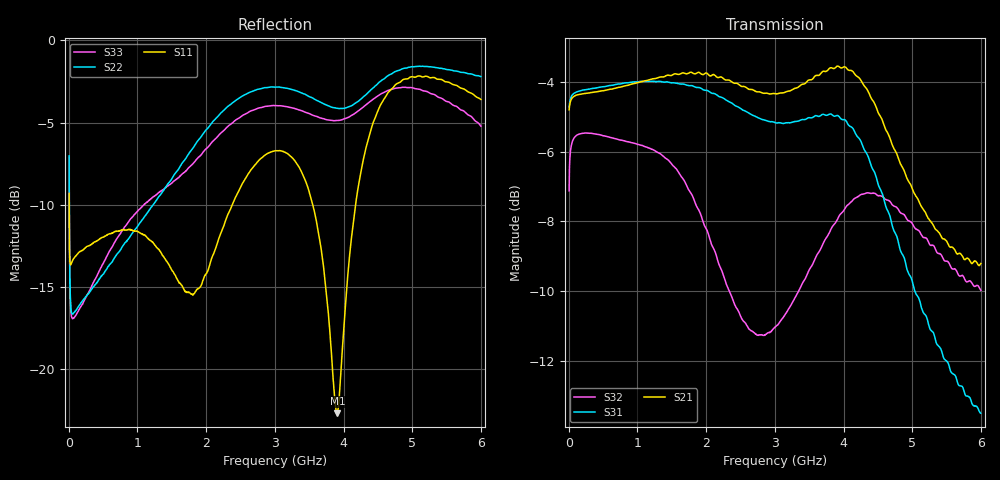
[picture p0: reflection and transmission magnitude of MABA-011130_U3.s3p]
!Agilent Technologies,E5071C,MY46110647,A.11.31
!Date: Fri Mar 25 10:46:57 2022 DD
!Data & Calibration Information:
!MABA-011130 soldered onto PT-0028476 with SMA connectors, Calibration PCB, Port1 (pin1) Port2 (pin2) Port3 (pin3)
!Freq	S11:SOLT3(ON)	S12:SOLT3(ON)	S13:SOLT3(ON)
!	S21:SOLT3(ON)	S22:SOLT3(ON)	S23:SOLT3(ON)
!	S31:SOLT3(ON)	S32:SOLT3(ON)	S33:SOLT3(ON)
!PortZ  Port1:50+j0  Port2:50+j0  Port3:50+j0
!Above PortZ is port z conversion or system Z0 setting when saving the data.
!When reading, reference impedance value at option line is always used.
# Hz S MA R 50
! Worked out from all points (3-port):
!   1200 points, 5 MHz to 6 GHz, reference 50 ohm
!   strongest paths, dB at 5 MHz, 1.505 GHz, 3.005 GHz, 4.505 GHz, 6 GHz:
!     S21: -4.8, -3.8, -4.3, -4.9, -9.2
!     S31: -4.7, -4.0, -5.2, -6.9, -13.5
!     S32: -7.1, -6.4, -11.0, -7.3, -10.0
!   lowest |S11| = -22.7 dB at 3.91 GHz (marker M1), VSWR 1.16, Z = 45.9 - j5.72 ohm
!   |S11| at or under -10 dB: 6.048 MHz to 2.379 GHz (2.373 GHz wide, 199 % of centre); 3.551 GHz to 4.175 GHz (623.6 MHz wide, 16.1 % of centre)
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5000000  0.3428 70.5  0.5701 -163.9  0.5751 15.6
         0.5749 -163.9  0.4456 103.0  0.4397 37.6
         0.58 15.6  0.4404 37.6  0.4396 102.8
7e7  0.2171 2.7  0.6008 176.6  0.6065 -3.2
     0.6004 176.6  0.1483 22.5  0.5226 1.1
     0.6065 -3.2  0.5227 1.1  0.1434 19.0
1.28e9  0.2344 -125.3  0.641 79.4  0.6291 -97.6
        0.6381 79.9  0.328 -65.3  0.5032 -67.6
        0.6311 -98.5  0.5004 -67.1  0.3402 -96.1
2.12e9  0.2279 -101.1  0.6409 9.9  0.6054 -167.0
        0.6451 10.5  0.5728 -99.8  0.3638 -114.4
        0.6065 -167.0  0.3622 -114.0  0.4988 -120.2
3.005e9  0.4615 -135.6  0.6099 -58.1  0.5508 122.4
         0.6062 -58.9  0.7209 -141.2  0.2887 -132.6
         0.5512 122.0  0.2814 -133.8  0.6336 -152.8
3.565e9  0.3081 -171.6  0.6511 -103.1  0.5616 74.0
         0.639 -103.2  0.665 -151.9  0.3563 -154.9
         0.5618 74.6  0.3484 -155.8  0.5908 -161.7
3.91e9  0.07356 -122.5  0.6685 -134.6  0.5564 40.3
        0.6636 -134.8  0.622 -148.1  0.4076 -176.4
        0.5643 40.5  0.4006 -177.0  0.5709 -158.2
4.215e9  0.3589 -79.7  0.6461 -164.1  0.5218 8.5
         0.6402 -164.6  0.6529 -140.8  0.4361 161.3
         0.5247 8.4  0.4326 161.1  0.6108 -153.4
4.685e9  0.7063 -115.4  0.5244 155.2  0.4038 -36.1
         0.5205 155.0  0.7884 -141.5  0.4203 127.8
         0.402 -36.1  0.4241 127.9  0.7087 -158.1
6e9  0.6615 169.4  0.3293 84.3  0.2081 -113.8
     0.3467 83.3  0.7758 171.5  0.3143 57.9
     0.2117 -112.8  0.3173 58.4  0.5486 141.6
